| IBIS file stm32u375_385_ufbga64_smps.ibs
[IBIS ver] 4.2
[File name] stm32u375_385_ufbga64_smps.ibs
[File Rev] 1.2
[Date] 23-06-2025
[Source] Data Created at STMicroelectronics
[Notes]  File originated from ELDO simulations.
[Disclaimer]  This information is for modeling purpose only and is
   not guaranted. The information is subject to change without
   notice.
[Copyright] Copyright 2025  STMicroelectronics Inc.
|   Component stm32u375_385_ufbga64_smps
[Component] stm32u375_385_ufbga64_smps
[Manufacturer] STMicroelectronics
[Package]
| variable   typ   min   max
R_pkg  0  NA  NA
L_pkg  0  NA  NA
C_pkg  0  NA  NA
[Pin]   signal_name   model_name
A1  VDD  power
A2  VDD11  nc
A3  PH3-BOOT0  io8_ft_100m_hslv
A4  PB6  io8_ft_100m_hslv
A5  PB3  io8_ft_100m_hslv
A6  PD2  io8_ft_100m_hslv
A7  PC10  io8_ft_100m_hslv
A8  VDD  power
B1  VBAT  power
B2  VSS  gnd
B3  PC13  io8_ft_100m_v33
B4  PB4  io8_ft_100m_hslv
B5  PC11  io8_ft_100m_hslv
B6  PC12  io8_ft_100m_hslv
B7  VSS  gnd
B8  VDDUSB  power
C1  PC14-OSC32_IN  io_ft_tamp
C2  PC15-OSC32_OUT  io_ft_tamp
C3  PB8  io8_ft_100m_hslv
C4  PA15  io8_ft_100m
C5  PA14  io8_ft_100m
C6  PA13  io8_ft_100m
C7  PA12  io8usb_ft_phy
C8  PA11  io8usb_ft_phy
D1  PH0-OSC_IN  io8_ft_100m
D2  PH1-OSC_OUT  io8_ft_100m
D3  PB7  io8_ft_100m_hslv
D4  PB5  io8_ft_100m_hslv
D5  PA10  io8_ft_100m
D6  PA9  io8_ft_100m
D7  PA8  io8_ft_100m_hslv
D8  PC9  io8_ft_100m_hslv
E1  NRST  ioreset_v33
E2  PC0  io8_ft_100m_hslv
E3  PC1  io8_ft_100m_hslv
E4  PC2  io8_ft_100m_hslv
E5  PA0  io8_ft_100m
E6  PB14  io8_ft_100m_hslv
E7  PC7  io8_ft_100m_hslv
E8  PC8  io8_ft_100m_hslv
F1  VSSA  nc
F2  PC3  io8_ft_100m_hslv
F3  PA1  io8_ft_100m_hslv
F4  PA4  io8_ft_100m_hslv
F5  PA6  io8_ft_100m_hslv
F6  PB10  io8_ft_100m_hslv
F7  PB15  io8_ft_100m
F8  PC6  io8_ft_100m_hslv
G1  VDDA  nc
G2  PA2  io8_ft_100m_hslv
G3  PA5  io8_ft_100m
G4  PB2  io8_ft_100m_hslv
G5  PB1  io8_ft_100m_hslv
G6  VSSSMPS  nc
G7  VSS  gnd
G8  PB13  io8_ft_100m_hslv
H1  VDD  power
H2  PA3  io8_ft_100m_hslv
H3  PA7  io8_ft_100m_hslv
H4  PB0  io8_ft_100m_hslv
H5  VLXSMPS  nc
H6  VDDSMPS  nc
H7  VDD11  nc
H8  VDD  power
[Package Model]   454-ufbga-5x5-64-smps-250417
[Pin Mapping]   pulldown_ref   pullup_ref   | Comment
A1  nc  vddio
A2  nc  nc
A3  gndio  vddio
A4  gndio  vddio
A5  gndio  vddio
A6  gndio  vddio
A7  gndio  vddio
A8  nc  vddio
B1  nc  vsw
B2  gndio  nc
B3  gndio  vsw
B4  gndio  vddio
B5  gndio  vddio
B6  gndio  vddio
B7  gndio  nc
B8  nc  vddusb
C1  gndio  vsw
C2  gndio  vsw
C3  gndio  vddio
C4  gndio  vddio
C5  gndio  vddio
C6  gndio  vddio
C7  gndio  vddusb  | Depending on IO usage
| C7  gndio  vddio  | Depending on IO usage
C8  gndio  vddusb  | Depending on IO usage
| C8  gndio  vddio  | Depending on IO usage
D1  gndio  vddio
D2  gndio  vddio
D3  gndio  vddio
D4  gndio  vddio
D5  gndio  vddio
D6  gndio  vddio
D7  gndio  vddio
D8  gndio  vddio
E1  gndio  vddio
E2  gndio  vddio
E3  gndio  vddio
E4  gndio  vddio
E5  gndio  vddio
E6  gndio  vddio
E7  gndio  vddio
E8  gndio  vddio
F1  nc  nc
F2  gndio  vddio
F3  gndio  vddio
F4  gndio  vddio
F5  gndio  vddio
F6  gndio  vddio
F7  gndio  vddio
F8  gndio  vddio
G1  nc  nc
G2  gndio  vddio
G3  gndio  vddio
G4  gndio  vddio
G5  gndio  vddio
G6  nc  nc
G7  gndio  nc
G8  gndio  vddio
H1  nc  vddio
H2  gndio  vddio
H3  gndio  vddio
H4  gndio  vddio
H5  nc  nc
H6  nc  nc
H7  nc  nc
H8  nc  vddio
|[Diff Pin]  inv_pin  vdiff  tdelay_typ  tdelay_min  tdelay_max
|C7  C8  NA  NA  NA  NA
[Model Selector] io8_ft_100m
io8_ft_100m_ls_1v2  "GPIO 100MHz - 5V tolerant - low speed - 1.2V range"
io8_ft_100m_ls_1v8  "GPIO 100MHz - 5V tolerant - low speed - 1.8V range"
io8_ft_100m_ls_3v3  "GPIO 100MHz - 5V tolerant - low speed - 3.3V range"
io8_ft_100m_ms_1v2  "GPIO 100MHz - 5V tolerant - med speed - 1.2V range"
io8_ft_100m_ms_1v8  "GPIO 100MHz - 5V tolerant - med speed - 1.8V range"
io8_ft_100m_ms_3v3  "GPIO 100MHz - 5V tolerant - med speed - 3.3V range"
io8_ft_100m_fs_1v2  "GPIO 100MHz - 5V tolerant - fast speed - 1.2V range"
io8_ft_100m_fs_1v8  "GPIO 100MHz - 5V tolerant - fast speed - 1.8V range"
io8_ft_100m_fs_3v3  "GPIO 100MHz - 5V tolerant - fast speed - 3.3V range"
io8_ft_100m_hs_1v2  "GPIO 100MHz - 5V tolerant - high speed - 1.2V range"
io8_ft_100m_hs_1v8  "GPIO 100MHz - 5V tolerant - high speed - 1.8V range"
io8_ft_100m_hs_3v3  "GPIO 100MHz - 5V tolerant - high speed - 3.3V range"
[Model Selector] io8_ft_100m_hslv
io8_ft_100m_ls_1v2  "GPIO 100MHz - 5V tolerant - low speed - 1.2V range"
io8_ft_100m_ls_1v8  "GPIO 100MHz - 5V tolerant - low speed - 1.8V range"
io8_ft_100m_ls_3v3  "GPIO 100MHz - 5V tolerant - low speed - 3.3V range"
io8_ft_100m_ms_1v2  "GPIO 100MHz - 5V tolerant - med speed - 1.2V range"
io8_ft_100m_ms_1v8  "GPIO 100MHz - 5V tolerant - med speed - 1.8V range"
io8_ft_100m_ms_3v3  "GPIO 100MHz - 5V tolerant - med speed - 3.3V range"
io8_ft_100m_fs_1v2  "GPIO 100MHz - 5V tolerant - fast speed - 1.2V range"
io8_ft_100m_fs_1v8  "GPIO 100MHz - 5V tolerant - fast speed - 1.8V range"
io8_ft_100m_fs_3v3  "GPIO 100MHz - 5V tolerant - fast speed - 3.3V range"
io8_ft_100m_hs_1v2  "GPIO 100MHz - 5V tolerant - high speed - 1.2V range"
io8_ft_100m_hs_1v8  "GPIO 100MHz - 5V tolerant - high speed - 1.8V range"
io8_ft_100m_hs_3v3  "GPIO 100MHz - 5V tolerant - high speed - 3.3V range"
io8_ft_100m_hslv_ls_1v2  "GPIO 100MHz low voltage optimization - 5V tolerant - low speed - 1.2V range"
io8_ft_100m_hslv_ls_1v8  "GPIO 100MHz low voltage optimization - 5V tolerant - low speed - 1.8V range"
io8_ft_100m_hslv_ls_2v5  "GPIO 100MHz low voltage optimization - 5V tolerant - low speed - 3.3V range"
io8_ft_100m_hslv_ms_1v2  "GPIO 100MHz low voltage optimization - 5V tolerant - med speed - 1.2V range"
io8_ft_100m_hslv_ms_1v8  "GPIO 100MHz low voltage optimization - 5V tolerant - med speed - 1.8V range"
io8_ft_100m_hslv_ms_2v5  "GPIO 100MHz low voltage optimization - 5V tolerant - med speed - 3.3V range"
io8_ft_100m_hslv_fs_1v2  "GPIO 100MHz low voltage optimization - 5V tolerant - fast speed - 1.2V range"
io8_ft_100m_hslv_fs_1v8  "GPIO 100MHz low voltage optimization - 5V tolerant - fast speed - 1.8V range"
io8_ft_100m_hslv_fs_2v5  "GPIO 100MHz low voltage optimization - 5V tolerant - fast speed - 3.3V range"
io8_ft_100m_hslv_hs_1v2  "GPIO 100MHz low voltage optimization - 5V tolerant - high speed - 1.2V range"
io8_ft_100m_hslv_hs_1v8  "GPIO 100MHz low voltage optimization - 5V tolerant - high speed - 1.8V range"
io8_ft_100m_hslv_hs_2v5  "GPIO 100MHz low voltage optimization - 5V tolerant - high speed - 3.3V range"
[Model Selector] io8_ft_100m_v33
io8_ft_100m_v33_ls_1v2  "GPIO_V33 100MHz - 5V tolerant - low speed - 1.2V range"
io8_ft_100m_v33_ls_1v8  "GPIO_V33 100MHz - 5V tolerant - low speed - 1.8V range"
io8_ft_100m_v33_ls_3v3  "GPIO_V33 100MHz - 5V tolerant - low speed - 3.3V range"
io8_ft_100m_v33_ms_1v2  "GPIO_V33 100MHz - 5V tolerant - med speed - 1.2V range"
io8_ft_100m_v33_ms_1v8  "GPIO_V33 100MHz - 5V tolerant - med speed - 1.8V range"
io8_ft_100m_v33_ms_3v3  "GPIO_V33 100MHz - 5V tolerant - med speed - 3.3V range"
io8_ft_100m_v33_fs_1v2  "GPIO_V33 100MHz - 5V tolerant - fast speed - 1.2V range"
io8_ft_100m_v33_fs_1v8  "GPIO_V33 100MHz - 5V tolerant - fast speed - 1.8V range"
io8_ft_100m_v33_fs_3v3  "GPIO_V33 100MHz - 5V tolerant - fast speed - 3.3V range"
io8_ft_100m_v33_hs_1v2  "GPIO_V33 100MHz - 5V tolerant - high speed - 1.2V range"
io8_ft_100m_v33_hs_1v8  "GPIO_V33 100MHz - 5V tolerant - high speed - 1.8V range"
io8_ft_100m_v33_hs_3v3  "GPIO_V33 100MHz - 5V tolerant - high speed - 3.3V range"
[Model Selector] io8usb_ft_phy
io8_ft_100m_ls_1v2  "GPIO 100MHz - 5V tolerant - low speed - 1.2V range"
io8_ft_100m_ls_1v8  "GPIO 100MHz - 5V tolerant - low speed - 1.8V range"
io8_ft_100m_ls_3v3  "GPIO 100MHz - 5V tolerant - low speed - 3.3V range"
io8_ft_100m_ms_1v2  "GPIO 100MHz - 5V tolerant - med speed - 1.2V range"
io8_ft_100m_ms_1v8  "GPIO 100MHz - 5V tolerant - med speed - 1.8V range"
io8_ft_100m_ms_3v3  "GPIO 100MHz - 5V tolerant - med speed - 3.3V range"
io8_ft_100m_fs_1v2  "GPIO 100MHz - 5V tolerant - fast speed - 1.2V range"
io8_ft_100m_fs_1v8  "GPIO 100MHz - 5V tolerant - fast speed - 1.8V range"
io8_ft_100m_fs_3v3  "GPIO 100MHz - 5V tolerant - fast speed - 3.3V range"
io8_ft_100m_hs_1v2  "GPIO 100MHz - 5V tolerant - high speed - 1.2V range"
io8_ft_100m_hs_1v8  "GPIO 100MHz - 5V tolerant - high speed - 1.8V range"
io8_ft_100m_hs_3v3  "GPIO 100MHz - 5V tolerant - high speed - 3.3V range"
io8usb_ft_phy_hs_3v3   "USB full speed"
io8usb_ft_phy_ls_3v3   "USB low speed"
[Model Selector] io_ft_tamp
io_ft_tamp_ls_1v2 "io8_ft tamp low speed @ 1.2V"
io_ft_tamp_ls_1v8 "io8_ft tamp low speed @ 1.8V"
io_ft_tamp_ls_3v3 "io8_ft tamp low speed @ 3.3V"
io_ft_tamp_ms_1v2 "io8_ft tamp med speed @ 1.2V"
io_ft_tamp_ms_1v8 "io8_ft tamp med speed @ 1.8V"
io_ft_tamp_ms_3v3 "io8_ft tamp med speed @ 3.3V"
io_ft_tamp_fs_1v2 "io8_ft tamp fast speed @ 1.2V"
io_ft_tamp_fs_1v8 "io8_ft tamp fast speed @ 1.8V"
io_ft_tamp_fs_3v3 "io8_ft tamp fast speed @ 3.3V"
io_ft_tamp_hs_1v2 "io8_ft tamp high speed @ 1.2V"
io_ft_tamp_hs_1v8 "io8_ft tamp high speed @ 1.8V"
io_ft_tamp_hs_3v3 "io8_ft tamp high speed @ 3.3V"
[Model Selector] ioreset_v33
ioreset_v33_1v2 "Reset PAD. 5V tolerant. 1.2V range"
ioreset_v33_1v8 "Reset PAD. 5V tolerant. 1.8V range"
ioreset_v33_3v3 "Reset PAD. 5V tolerant. 3.3V range"
[Define Package Model]  454-ufbga-5x5-64-smps-250417
[Manufacturer]  unknown
[OEM]  unknown
[Description]  unknown
[Number Of Pins]  59
[Pin Numbers]
| Pin Name Terminal   Net Name   Starting Node   Ending Node
E1 | NRST
E5 | PA0
F3 | PA1
G2 | PA2
H2 | PA3
F4 | PA4
G3 | PA5
F5 | PA6
H3 | PA7
D7 | PA8
D6 | PA9
D5 | PA10
C8 | PA11
C7 | PA12
C6 | PA13
C5 | PA14
C4 | PA15
H4 | PB0
G5 | PB1
G4 | PB2
A5 | PB3
B4 | PB4
D4 | PB5
A4 | PB6
D3 | PB7
C3 | PB8
F6 | PB10
G8 | PB13
E6 | PB14
F7 | PB15
E2 | PC0
E3 | PC1
E4 | PC2
F2 | PC3
F8 | PC6
E7 | PC7
E8 | PC8
D8 | PC9
A7 | PC10
B5 | PC11
B6 | PC12
B3 | PC13
C1 | PC14-OSC32_IN
C2 | PC15-OSC32_OUT
A6 | PD2
D1 | PH0-OSC_IN
D2 | PH1-OSC_OUT
A3 | PH3-BOOT0
H7 | VDD11
A2 | VDD11
B1 | VBAT
A1 | VDD
G1 | VDDA
H6 | VDDSMPS
B8 | VDDUSB
H5 | VLXSMPS
B2 | VSS
F1 | VSSA
G6 | VSSSMPS
|[Merged Pins]  A1
|A8  |  VDD
|H1  |  VDD
|H8  |  VDD
|[Merged Pins]  B2
|B7  |  VSS
|G7  |  VSS
[Model Data]
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[End Model Data]
[End Package Model]
|End [Component]
| Models and submodels in the file (53): io8_ft_100m_fs_1v2 (I/O), io8_ft_100m_fs_1v8 (I/O), io8_ft_100m_fs_3v3 (I/O), io8_ft_100m_hs_1v2 (I/O), io8_ft_100m_hs_1v8 (I/O), io8_ft_100m_hs_3v3 (I/O), io8_ft_100m_hslv_fs_1v2 (I/O), io8_ft_100m_hslv_fs_1v8 (I/O), io8_ft_100m_hslv_fs_2v5 (I/O), io8_ft_100m_hslv_hs_1v2 (I/O), io8_ft_100m_hslv_hs_1v8 (I/O), io8_ft_100m_hslv_hs_2v5 (I/O), io8_ft_100m_hslv_ls_1v2 (I/O), io8_ft_100m_hslv_ls_1v8 (I/O), io8_ft_100m_hslv_ls_2v5 (I/O), io8_ft_100m_hslv_ms_1v2 (I/O), io8_ft_100m_hslv_ms_1v8 (I/O), io8_ft_100m_hslv_ms_2v5 (I/O), io8_ft_100m_ls_1v2 (I/O), io8_ft_100m_ls_1v8 (I/O), io8_ft_100m_ls_3v3 (I/O), io8_ft_100m_ms_1v2 (I/O), io8_ft_100m_ms_1v8 (I/O), io8_ft_100m_ms_3v3 (I/O), io8_ft_100m_v33_fs_1v2 (I/O), io8_ft_100m_v33_fs_1v8 (I/O), io8_ft_100m_v33_fs_3v3 (I/O), io8_ft_100m_v33_hs_1v2 (I/O), io8_ft_100m_v33_hs_1v8 (I/O), io8_ft_100m_v33_hs_3v3 (I/O), io8_ft_100m_v33_ls_1v2 (I/O), io8_ft_100m_v33_ls_1v8 (I/O), io8_ft_100m_v33_ls_3v3 (I/O), io8_ft_100m_v33_ms_1v2 (I/O), io8_ft_100m_v33_ms_1v8 (I/O), io8_ft_100m_v33_ms_3v3 (I/O), io8usb_ft_phy_hs_3v3 (I/O), io8usb_ft_phy_ls_3v3 (I/O), io_ft_tamp_fs_1v2 (I/O), io_ft_tamp_fs_1v8 (I/O), io_ft_tamp_fs_3v3 (I/O), io_ft_tamp_hs_1v2 (I/O), io_ft_tamp_hs_1v8 (I/O), io_ft_tamp_hs_3v3 (I/O), io_ft_tamp_ls_1v2 (I/O), io_ft_tamp_ls_1v8 (I/O), io_ft_tamp_ls_3v3 (I/O), io_ft_tamp_ms_1v2 (I/O), io_ft_tamp_ms_1v8 (I/O), io_ft_tamp_ms_3v3 (I/O), ioreset_v33_1v2 (I/O_open_drain), ioreset_v33_1v8 (I/O_open_drain), ioreset_v33_3v3 (I/O_open_drain)
